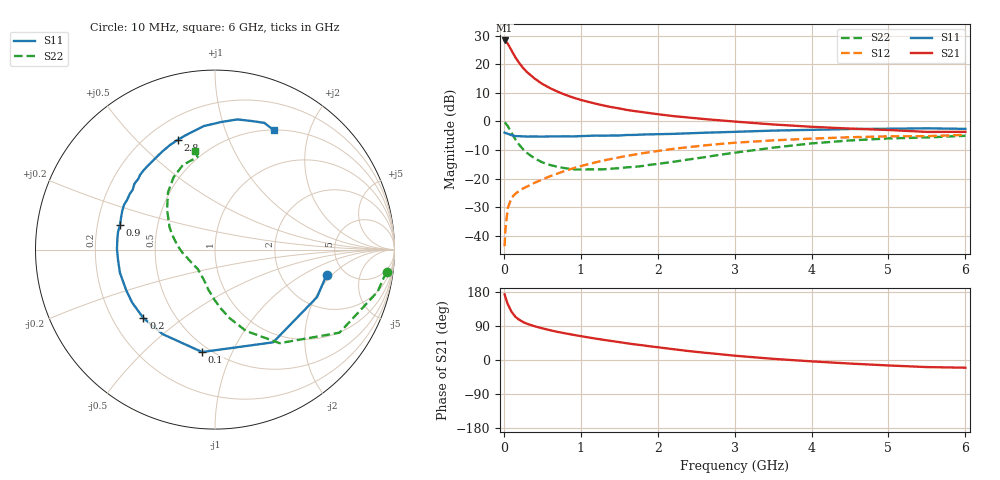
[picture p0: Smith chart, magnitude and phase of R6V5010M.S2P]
! SIEMENS Small Signal Semiconductors
! BFR193
! Si NPN RF Bipolar Junction Transistor in SOT23
! VCE = 0.5 V  IC = 10 mA
! Common Emitter S-Parameters:  May  1996
# GHz  S  MA  R  50
!  f  S11  S21  S12  S22
! GHz  MAG  ANG  MAG  ANG  MAG  ANG  MAG  ANG
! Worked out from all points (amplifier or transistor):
!   36 points, 10 MHz to 6 GHz, reference 50 ohm
!   highest |S21| = 28.3 dB at 10 MHz (marker M1)
!   |S21| within 3 dB of that: start of sweep to 89.4 MHz
!   unconditionally stable (mu >= 1): 646.9 MHz to 2.521 GHz
!   at 250 MHz: K = 0.66, MSG = 21.1 dB, |S12| = -23.4 dB
!   at 1.4 GHz: K = 1.06, MAG = 7.5 dB, |S12| = -13.1 dB
!   at 6 GHz: K = 1.00, MSG = 0.5 dB, |S12| = -4.7 dB
!   S11 on the Smith chart (normalised r, x): 10 MHz: 3.64, -1.73; 100 MHz: 0.45, -0.77; 200 MHz: 0.33, -0.36; 900 MHz: 0.30, +0.12; 2.8 GHz: 0.32, +0.67; 6 GHz: 0.51, +1.49
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0.01  0.6375 -12.8  26.02 173.2  0.0066 84.1  0.9634 -7.3
0.02  0.6271 -25.0  25.71 166.0  0.0129 81.5  0.9359 -14.5
0.05  0.6098 -57.9  22.97 147.9  0.03 65.5  0.834 -33.7
0.1  0.5752 -97.2  17.35 127.2  0.0462 54.0  0.6335 -55.4
0.15  0.554 -121.8  13.2 114.1  0.0545 49.3  0.4842 -69.2
0.2  0.5521 -136.3  10.51 106.2  0.061 48.1  0.3901 -78.0
0.25  0.5478 -147.5  8.605 100.2  0.0673 48.6  0.3266 -84.7
0.3  0.5441 -155.2  7.311 95.7  0.0726 49.9  0.2819 -90.3
0.4  0.5452 -166.3  5.615 89.1  0.0845 52.2  0.2261 -99.4
0.5  0.5433 -173.7  4.527 83.6  0.0966 54.3  0.1924 -106.5
0.6  0.5463 179.8  3.82 78.7  0.11 55.3  0.1731 -112.7
0.7  0.547 174.2  3.309 74.1  0.1232 56.2  0.1607 -119.1
0.9  0.5469 165.6  2.616 66.5  0.1515 56.8  0.1458 -129.9
1.1  0.5601 157.3  2.195 59.5  0.1796 55.9  0.1451 -138.4
1.3  0.5626 150.3  1.894 53.1  0.208 54.5  0.1457 -147.3
1.6  0.5796 140.8  1.587 44.1  0.2499 51.5  0.1576 -159.8
2.2  0.6059 124.0  1.24 28.6  0.331 43.6  0.1967 178.9
2.8  0.6454 108.8  1.047 15.5  0.4027 34.5  0.26 159.1
3.5  0.691 95.2  0.885 3.1  0.4665 23.2  0.3477 140.2
4.5  0.736 80.2  0.75 -9.4  0.5291 9.1  0.465 119.7
5.5  0.7578 68.7  0.656 -18.7  0.5529 -4.1  0.525 100.7
6  0.7409 63.6  0.658 -20.3  0.5831 -8.1  0.5611 101.2
